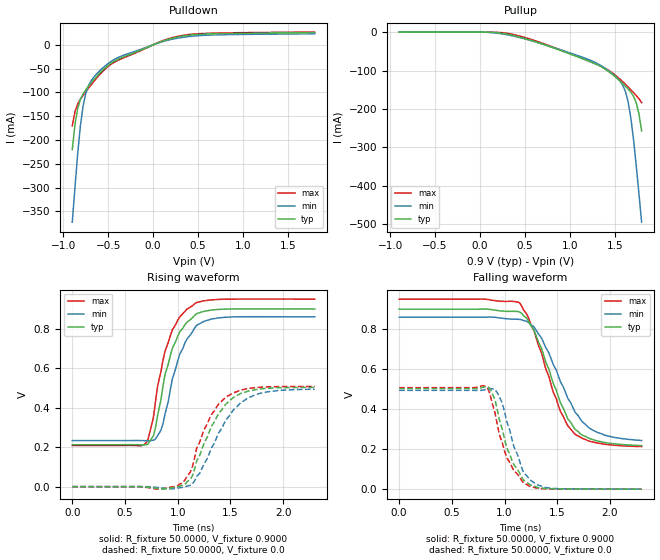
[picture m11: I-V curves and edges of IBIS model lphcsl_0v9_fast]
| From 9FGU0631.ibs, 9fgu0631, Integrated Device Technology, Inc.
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[Model]  lphcsl_0v9_fast
Model_type Output
Polarity   Non-Inverting
Enable   Active-High
Vmeas =  0.4000V
Cref =   2.0000pF
Rref =   0.0
Vref =   0.4000V
C_comp   1.1000pF   1.0000pF   1.2000pF
[Temperature Range]   25.0000   75.0000   0.0
[Voltage Range]   0.9000V   0.8600V   0.9500V
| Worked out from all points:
|   slope of the pulldown table from 0 to 0.135 V, typ, clamps not added: 14 ohm
|   slope of the pullup table from 0 to 0.135 V, typ, clamps not added: 242 ohm
|   rising waveform, R_fixture 50.0000, V_fixture 0.9000: 20-80 % time 195ps typ, 199ps min, 187ps max; typ from 0.212 V to 0.9 V
|   rising waveform, R_fixture 50.0000, V_fixture 0.0: 20-80 % time 269ps typ, 304ps min, 232ps max; typ from 0 V to 0.503 V
|   falling waveform, R_fixture 50.0000, V_fixture 0.9000: 20-80 % time 296ps typ, 333ps min, 290ps max; typ from 0.9 V to 0.218 V
|   falling waveform, R_fixture 50.0000, V_fixture 0.0: 20-80 % time 191ps typ, 173ps min, 184ps max; typ from 0.503 V to 0 V
[Pulldown]
|Voltage   I(typ)   I(min)   I(max)
-900mV    -219.9mA   -372.5mA   -170.2mA
-870mV    -167.7mA   -299.2mA   -140.4mA
-840mV    -134mA     -229.3mA   -124.2mA
-810mV    -114.7mA   -170.8mA   -114.3mA
-780mV    -103.1mA   -129mA     -106.3mA
-750mV    -94.51mA   -102.1mA   -98.78mA
-720mV    -87.03mA   -85.88mA   -91.35mA
-660mV    -73.27mA   -67.73mA   -76.97mA
-510mV    -44.58mA   -40.66mA   -46.85mA
60mV      4.726mA    3.957mA    5.199mA
330mV     18.28mA    15.74mA    19.79mA
1.8V      25.49mA    23.19mA    26.76mA
[Pullup]
|Voltage   I(typ)   I(min)   I(max)
-900mV    58.12uA    179.8uA    108.4uA
30mV      -27.1uA    -120.7uA   -3.07uA
330mV     -6.434mA   -8.091mA   -4.143mA
1.17V     -71.69mA   -67.79mA   -71.08mA
1.47V     -109.4mA   -107.2mA   -105.3mA
1.59V     -134.1mA   -138.1mA   -129.1mA
1.62V     -141mA     -154.8mA   -135.9mA
1.65V     -148.2mA   -181.8mA   -142.9mA
1.68V     -156.4mA   -223.1mA   -150.2mA
1.74V     -183.8mA   -347.1mA   -165.1mA
1.77V     -212.4mA   -420.1mA   -173.2mA
1.8V      -256.9mA   -494.7mA   -183.7mA
[Ramp]
| variable   typ   min   max
dV/dt_r  0.3016/0.2694n   0.2960/0.2999n   0.3045/0.2559n
dV/dt_f  0.4094/0.2942n   0.3700/0.3258n   0.4423/0.2839n
R_load = 50.0000
[Rising Waveform]
R_fixture= 50.0000
V_fixture= 0.9000
V_fixture_min= 0.8600
V_fixture_max= 0.9500
|time   V(typ)   V(min)   V(max)
0s        212.3mV    233.4mV    208.8mV
700ps     212.1mV    232.6mV    220.4mV
770ps     257.1mV    235.2mV    351.7mV
840ps     437.7mV    284.7mV    580.4mV
880ps     568.7mV    369mV      686.6mV
950ps     701.8mV    546.8mV    795mV
1.02ns    784.8mV    672.4mV    860mV
1.18ns    876.1mV    817.3mV    932.8mV
1.46ns    899.3mV    858.2mV    949.5mV
2.3ns     899.9mV    860mV      949.9mV
[Rising Waveform]
R_fixture= 50.0000
V_fixture= 0.0
V_fixture_min= 0.0
V_fixture_max= 0.0
|time   V(typ)   V(min)   V(max)
0s        0V         0V         0V
840ps     -11.93mV   -6.086mV   -11.87mV
1.05ns    7.731mV    -3.369mV   19.57mV
1.12ns    37.27mV    6.688mV    74.33mV
1.18ns    130mV      51.56mV    194.7mV
1.25ns    220.3mV    115.7mV    289.1mV
1.46ns    420mV      339.6mV    455.7mV
1.6ns     472.8mV    426.6mV    489.2mV
1.74ns    491.4mV    466.1mV    502mV
2.3ns     502.6mV    493.3mV    507.5mV
[Falling Waveform]
R_fixture= 50.0000
V_fixture= 0.9000
V_fixture_min= 0.8600
V_fixture_max= 0.9500
|time   V(typ)   V(min)   V(max)
0s        900mV      860mV      950mV
1.14ns    886.6mV    849mV      933mV
1.21ns    855.2mV    839.3mV    875.3mV
1.35ns    705mV      756mV      682.2mV
1.46ns    530.7mV    625.1mV    487.5mV
1.53ns    431.9mV    537.3mV    388.8mV
1.63ns    332.1mV    429.4mV    298.1mV
1.74ns    269.5mV    335.2mV    253.1mV
1.84ns    247.5mV    294.5mV    235.8mV
2.3ns     217.7mV    243.4mV    212.8mV
[Falling Waveform]
R_fixture= 50.0000
V_fixture= 0.0
V_fixture_min= 0.0
V_fixture_max= 0.0
|time   V(typ)   V(min)   V(max)
0s        502.9mV    494.1mV    507.7mV
790ps     508.3mV    494.7mV    517.4mV
860ps     504.7mV    501.3mV    478.5mV
910ps     446.1mV    498.2mV    380.6mV
950ps     348.5mV    462.7mV    274.1mV
1.02ns    206.4mV    339.6mV    157.7mV
1.18ns    44.7mV     82.81mV    30.95mV
1.23ns    26.85mV    53.99mV    16.58mV
1.44ns    2.216mV    4.834mV    1.627mV
2.3ns     95.98uV    174.7uV    67.74uV
